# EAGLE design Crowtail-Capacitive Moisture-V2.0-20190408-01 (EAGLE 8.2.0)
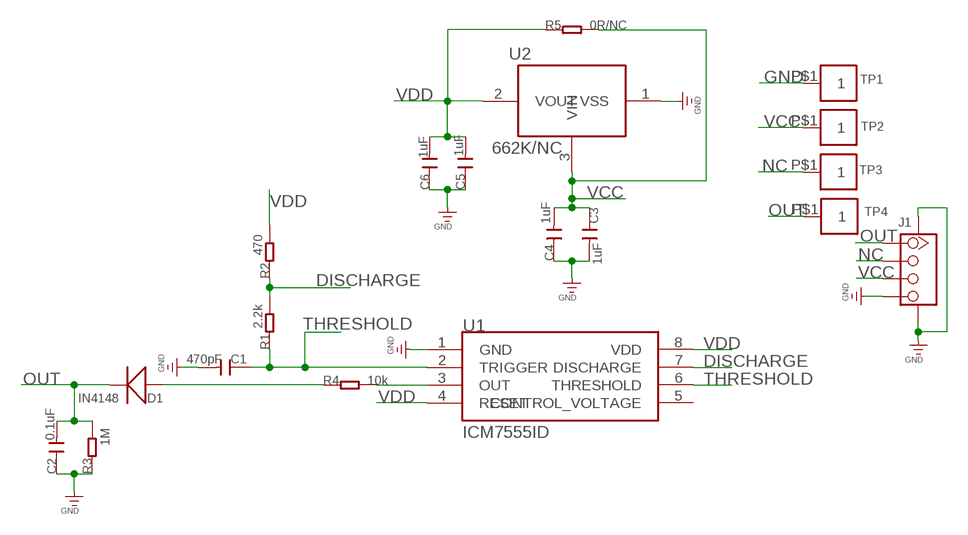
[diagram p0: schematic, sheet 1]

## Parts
C1  470pF  DISCRETE_C-0603  [DISCRETE_C0603]
C2  0.1uF  DISCRETE_C-0603  [DISCRETE_C0603]
C3  1uF  DISCRETE_C-0603  [DISCRETE_C0603]
C4  1uF  DISCRETE_C-0603  [DISCRETE_C0603]
C5  1uF  DISCRETE_C-0603  [DISCRETE_C0603]
C6  1uF  DISCRETE_C-0603  [DISCRETE_C0603]
D1  IN4148  DISCRETE_D1N4148-SMD  [DISCRETE_1206-1]
J1  TWIG-4P-2.0-SMD-FEMALE-REINFORCE'90D'  [4P-SMD-2.0-90D]
R1  2.2k  DISCRETE_R-0603  [DISCRETE_R0603]
R2  470  DISCRETE_R-0603  [DISCRETE_R0603]
R3  1M  DISCRETE_R-0603  [DISCRETE_R0603]
R4  10k  DISCRETE_R-0603  [DISCRETE_R0603]
R5  0R/NC  DISCRETE_R-0603  [DISCRETE_R0603]
TP1  COOPER_PAD1.2X2  [COOPER_PAD1.2X2]
TP2  COOPER_PAD1.2X2  [COOPER_PAD1.2X2]
TP3  COOPER_PAD1.2X2  [COOPER_PAD1.2X2]
TP4  COOPER_PAD1.2X2  [COOPER_PAD1.2X2]
U1  ICM7555ID  7555ID  [SOP8]
U2  662K/NC  662K  [SOT23]

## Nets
DISCHARGE: R1.2 R2.1 U1.7(DISCHARGE)
GND: C1.2 C2.1 C3.2 C4.1 C5.1 C6.1 J1.4 J1.SS1 J1.SS2 R3.1 TP1.P$1 U1.1(GND) U2.1(VSS)
N$1: R4.2 U1.3(OUT)
N$4: D1.A(+) R4.1
NC: J1.2 TP3.P$1
OUT: C2.2 D1.C(-) J1.1 R3.2 TP4.P$1
THRESHOLD: C1.1 R1.1 U1.2(TRIGGER) U1.6(THRESHOLD)
VCC: C3.1 C4.2 J1.3 R5.2 TP2.P$1 U2.3(VIN)
VDD: C5.2 C6.2 R2.2 R5.1 U1.4(RESET) U1.8(VDD) U2.2(VOUT)
Unconnected: U1.5(CONTROL_VOLTAGE)

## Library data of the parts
C1-C6 = Crowtail-_PIR_Sensor_v1.0:DISCRETE_C*: Ceramic Capacitors
D1 = Crowtail-_Sound_Sensor_v1.0:DISCRETE_D*
J1 = Connector:TWIG-4P-2.0-SMD-FEMALE-REINFORCE
R1-R5 = Crowtail-_PIR_Sensor_v1.0:DISCRETE_R*
TP1-TP4 = Crowcube-Moisture_Sensor-V1.0-20181218-01:COOPER_PAD1.2X2
U1 = Lib:7555ID
U2 = Lib:662K

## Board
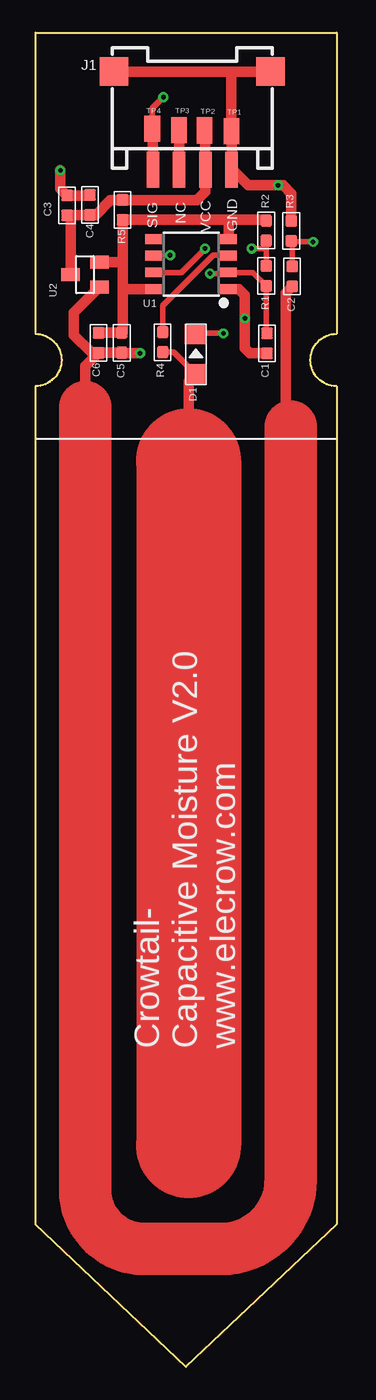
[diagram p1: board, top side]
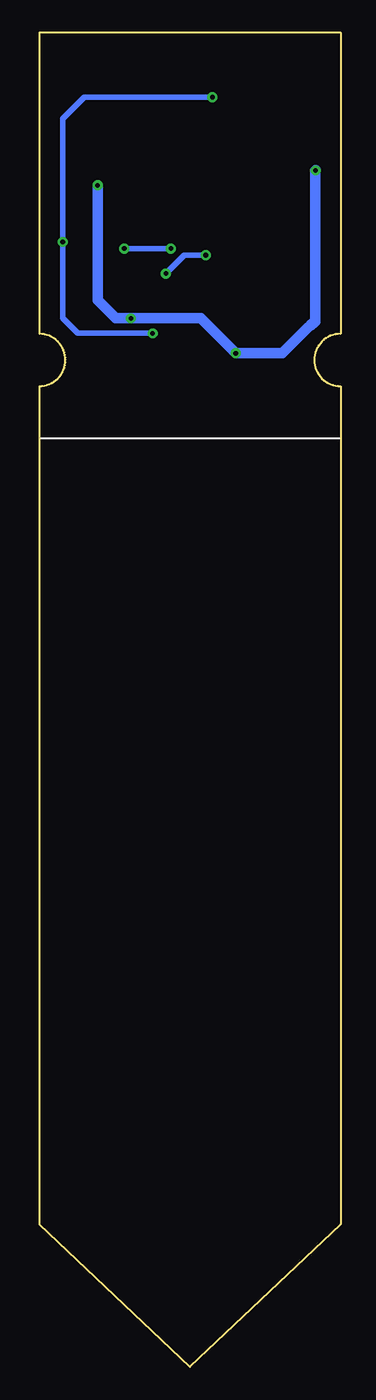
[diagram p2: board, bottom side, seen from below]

Size 23 x 101.9 mm. Coordinates in mm from the lower left corner, seen from the top.
Outline: 0,101.9 23,101.9 23,78.9 arc180 23,74.9 23,10.9 11.5,0 0,10.9 0,74.9 arc180 0,78.9 0,101.9
Copper layers (1*16): Top 0.035mm / dielectric 1.5mm / Bottom 0.035mm
Design rules "default *": minimum track width 8mil, minimum drill 10mil, track to track 8mil, track to pad 8mil, pad to pad 8mil, via to via 8mil, smd to smd 8mil, copper to edge 40mil, drill to drill 8mil, minimum pad ring 10mil, minimum via ring 8mil, stop-mask expansion 4mil, vias tented up to drill 100mil, thermal gap 10mil

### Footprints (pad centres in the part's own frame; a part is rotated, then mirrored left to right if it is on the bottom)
DISCRETE_C0603 = smd 0.889 x 0.889: 1 -0.762,0; 2 0.762,0
DISCRETE_1206-1 = smd 1.524 x 1.676: A -1.524,0; C 1.524,0
4P-SMD-2.0-90D = smd 0.965 x 2.74: 1 -3,-0.1; 2 -1,-0.1; 3 1,-0.1; 4 3,-0.1 | smd 2.159 x 2.184: SS1 -5.974,7.4; SS2 5.974,7.4
DISCRETE_R0603 = smd 0.889 x 0.889: 1 -0.762,0; 2 0.762,0
COOPER_PAD1.2X2 = smd 1.2 x 2: P$1 0,0
SOP8 = smd 0.76 x 1.27: 1 -1.905,-2.86; 2 -0.635,-2.86; 3 0.635,-2.86; 4 1.905,-2.86; 5 1.905,2.86; 6 0.635,2.86; 7 -0.635,2.86; 8 -1.905,2.86
SOT23 = smd 1 x 1.4: 1 -0.95,-1.1; 2 0.95,-1.1; 3 0,1.1

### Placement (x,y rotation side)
C1  17.69,78.17 270 top
C2  19.61,83.29 90 top
C3  2.41,88.71 90 top
C4  4.17,88.74 270 top
C5  6.59,78.22 90 top
C6  4.82,78.21 90 top
D1  12.26,77.34 90 top
J1  11.98,91.54 0 top
R1  17.63,83.33 90 top
R2  17.63,86.78 90 top
R3  19.54,86.75 270 top
R4  9.72,78.26 90 top
R5  6.66,88.37 90 top
TP1  14.97,94.38 0 top
TP2  12.92,94.44 0 top
TP3  10.97,94.46 0 top
TP4  8.92,94.56 0 top
U1  11.89,84.23 90 top
U2  3.79,83.42 90 top

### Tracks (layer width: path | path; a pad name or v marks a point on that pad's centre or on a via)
DISCHARGE  (via drill 0.35)
  Top 0.406: U1.7 11.13,83.59 v12.95,85.41 | 17.63,85.41 R1.2 | 17.63,85.41 R2.1 | v16.51,85.41 17.63,85.41
  Bottom 0.406: v12.95,85.41 v16.51,85.41
GND  (via drill 0.35)
  Top 0.813: C4.1 4.14,89.47 C3.2 1.91,89.98 v1.91,91.38 | 14.86,98.94 J1.SS1 | 14.86,98.94 J1.SS2 | J1.4 TP1.P$1 14.97,98.82 14.86,98.94 | C5.1 C6.1 | C5.1 | C6.1 4.29,77.45 2.95,78.79 2.95,80.53 U2.1 | 19.56,82.48 C2.1 19.1,82.02 19.1,73 19.61,72.49 19.61,71.92 arc-90 19.5,71.81 | J1.4 14.98,91.64 | J1.4 15.06,91.44 16.26,90.24 v18.54,90.24 18.92,90.24 19.56,89.61 19.56,87.53 R3.1 | v8,77.41 6.62,77.41 C5.1 | U1.1 15.54,82.32 16,81.86 v16,80.08 16,77.8 16.38,77.41 C1.2 | C6.1 3.8,76.43 3.8,73.3
  Top 4: 3.8,73.3 3.8,13.5 arc90 8.3,9 14.2,9 arc90 19.5,14.3 19.5,71.81
  Bottom 0.813: v18.54,90.24 18.54,81.48 17.14,80.08 v16,80.08 10.67,80.08 v8,77.41 4.45,77.41 2.48,79.38 2.33,79.52 2.01,79.78 1.91,79.84 v1.91,91.38
N$1
  Top 0.406: R4.2 9.72,81.04 13.59,84.91 14.7,84.91 U1.3
N$4
  Top 0.406: R4.1 10.58,77.5 D1.A
  Top 0.813: 12.2,75.76 D1.A 11.7,75.26 11.7,69.2
  Top 8: 11.7,69.2 11.7,16.9
NC
  Top 0.813: J1.2 TP3.P$1
OUT  (via drill 0.35)
  Top 0.406: 19.61,85.93 C2.2 | 19.61,85.93 R3.2 | TP4.P$1 8.92,96.12 v9.78,96.97 | v21.21,85.92 19.61,85.92 19.61,85.93 | v14.35,78.94 12.33,78.94 D1.C
  Top 0.813: J1.1 8.98,94.5 TP4.P$1
  Bottom 0.406: v9.78,96.97 19.56,96.97 21.21,95.32 v21.21,85.92 21.21,80.08 20.07,78.94 v14.35,78.94
THRESHOLD  (via drill 0.35)
  Top 0.406: C1.1 17.63,78.99 R1.1 16.61,83.59 U1.2 14.67,83.51 v13.34,83.51 | U1.6 10.24,84.86 v10.29,84.91
  Bottom 0.406: v10.29,84.91 11.94,84.91 v13.34,83.51
VCC
  Top 0.813: TP2.P$1 12.98,94.38 J1.3 12.98,89.76 12.32,89.1 6.69,89.1 R5.2 6.62,89.1 5.71,89.1 4.59,87.98 C4.2 4.14,87.95 C3.1 2.69,87.67 U2.3
VDD
  Top 0.813: 6.66,84.27 6.66,82.37 | 6.66,84.27 R5.1 14.73,87.61 | 6.66,82.37 6.66,79.05 C5.2 6.58,78.97 C6.2 | U1.8 6.7,82.32 6.66,82.37 | U2.2 6.56,84.37 6.66,84.27 | 14.73,87.61 17.57,87.61 R2.2 | U1.4 14.75,87.59 14.73,87.61

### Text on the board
tPlace: SIG | NC | VCC | GND | Crowtail- / Capacitive Moisture V2.0 / www.elecrow.com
